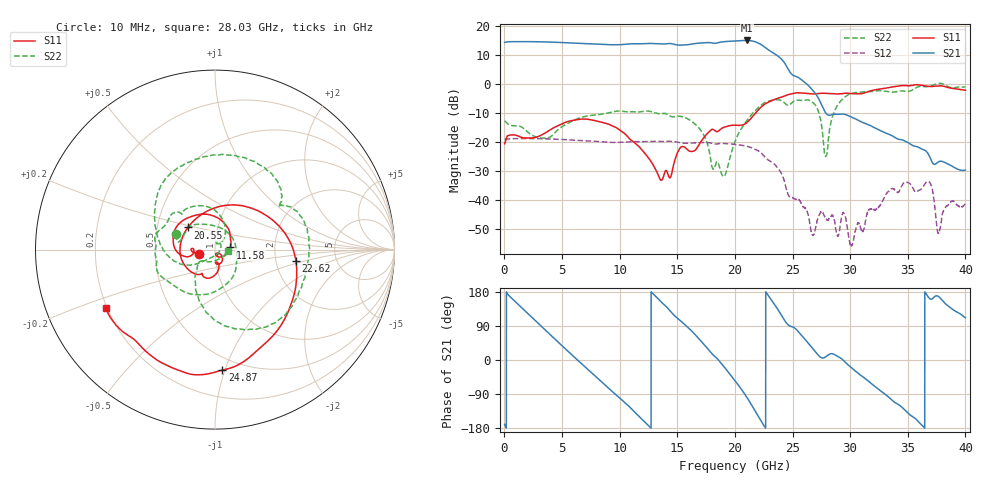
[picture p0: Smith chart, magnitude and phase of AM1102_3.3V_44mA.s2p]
!Agilent Technologies,E8364B,MY43040894,A.07.50.67
!Agilent E8364B: A.07.50.67
!Date: Thursday, June 11, 2020 10:43:29
!Correction: S11(Full 2 Port(1,2))
!S21(Full 2 Port(1,2))
!S12(Full 2 Port(1,2))
!S22(Full 2 Port(1,2))
!S2P File: Measurements: S11, S21, S12, S22:
# Hz S  dB  R 50
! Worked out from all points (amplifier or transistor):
!   6401 points, 10 MHz to 40 GHz, reference 50 ohm
!   highest |S21| = 15.0 dB at 21.04 GHz (marker M1)
!   |S21| within 3 dB of that: start of sweep to 22.82 GHz
!   unconditionally stable (mu >= 1): start of sweep to 37.46 GHz; 38.08 GHz to end of sweep
!   at 6.671 GHz: K = 1.14, MAG = 14.5 dB, |S12| = -19.5 dB
!   at 20 GHz: K = 1.21, MAG = 15.1 dB, |S12| = -20.8 dB
!   at 40 GHz: K = 148.36, MAG = -18.9 dB, |S12| = -41.3 dB
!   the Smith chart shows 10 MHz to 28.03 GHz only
!   S11 on the Smith chart (normalised r, x): 10 MHz: 0.83, -0.04; 11.58 GHz: 1.19, +0.03; 20.55 GHz: 0.72, +0.18; 22.62 GHz: 2.59, -0.41; 24.87 GHz: 0.40, -0.98; 28.03 GHz: 0.19, -0.24
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1e7  -20.57 -165.8  14.36 -169.9  -19.01 12.5  -12.69 158.6
1.622097e9  -18.53 179.3  14.62 134.2  -18.79 -37.8  -15.19 125.9
3.152964e9  -17.68 -167.1  14.55 90.3  -18.84 -74.9  -18.59 43.3
5.058738e9  -13.57 -175.8  14.29 35.8  -19.12 -121.0  -14.53 -61.1
6.677083e9  -12.08 156.5  13.99 -9.6  -19.49 -159.5  -11.51 -108.6
9.138967e9  -13.98 101.4  13.56 -77.6  -20.08 143.1  -9.86 -148.5
1.158211e10  -21.21 7.7  13.86 -145.9  -19.85 85.4  -9.63 176.0
1.334417e10  -31.40 -82.7  13.91 160.9  -19.76 40.1  -10.22 153.3
1.466259e10  -28.02 -39.5  13.76 119.8  -19.84 4.2  -11.33 132.9
1.65871e10  -22.67 -78.9  13.98 65.6  -20.23 -44.7  -13.98 84.2
1.864284e10  -15.93 -120.5  14.36 -2.7  -20.50 -105.1  -28.55 28.3
2.0005e10  -14.18 178.5  14.83 -54.5  -20.84 -152.2  -19.83 -137.5
2.054861e10  -14.20 140.7  14.97 -76.8  -21.08 -172.3  -15.44 -149.4
2.104224e10  -13.25 103.0  15.02 -98.9  -21.43 167.3  -12.51 -164.2
2.190452e10  -9.47 36.4  14.35 -142.2  -22.75 127.8  -8.59 154.3
2.26231e10  -6.85 -7.9  12.58 -178.0  -25.23 93.1  -6.30 124.2
2.380405e10  -4.77 -55.7  9.41 129.6  -29.42 35.7  -5.46 61.5
2.486628e10  -3.44 -86.5  3.64 88.6  -38.92 6.0  -6.71 32.6
2.667208e10  -3.40 -129.1  -1.78 33.1  -51.42 -163.0  -6.08 -63.5
2.803424e10  -3.21 -151.8  -10.56 12.3  -46.94 167.6  -22.49 -1.6
3.333917e10  -1.24 128.4  -17.28 -97.9  -36.92 -90.3  -2.63 168.3
4e10  -2.14 -13.1  -29.64 111.2  -41.28 78.0  -1.06 58.7
